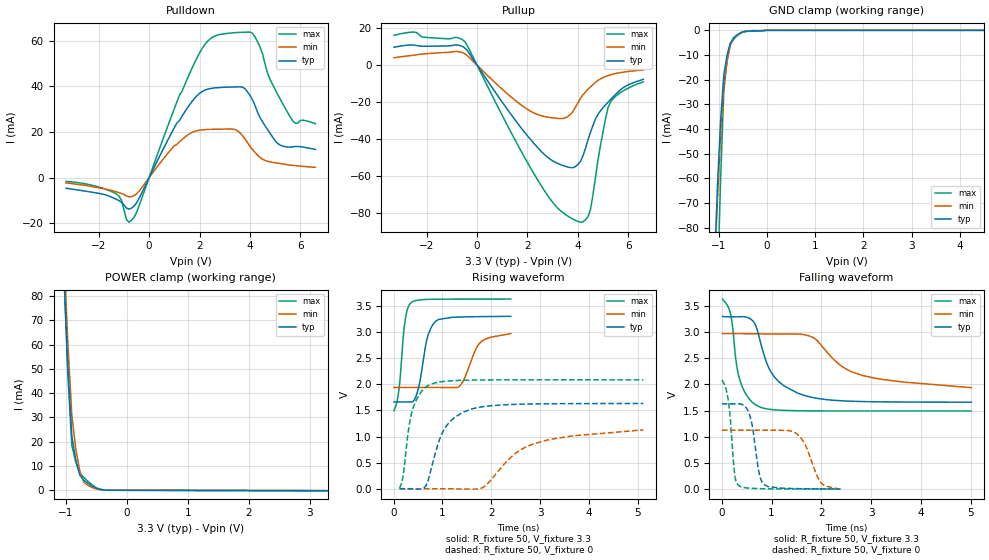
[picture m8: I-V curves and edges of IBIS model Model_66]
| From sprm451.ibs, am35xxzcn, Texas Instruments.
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| Model based on original model for BC1833DV50BTPBFHP18LL_7LM_X50
|   Sub model LL_7LM_X50_PU_ON_3P3
[model]   Model_66
|[Description]  3.3V-I/O-PU-X
|[Input Load]   PU
|[Output Drive]
|Voltage   3.3V
|Mode   I/O
Model_type   I/O
Polarity   Non-Inverting
Enable   Active-Low
Vinl =  0.8V
Vinh =  2V
Cref =  15pF
Rref =  100.0000M
Vref =  0V
Vmeas =  1.65
C_comp   1.683006p   1.492615p   1.787227p
[Model Spec]
Vinl   0.8V   0.8V   0.8V
Vinh   2V   2V   2V
[Temperature Range]   25   125   -40
[Voltage Range]   3.3   2.97   3.63
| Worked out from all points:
|   slope of the pulldown table from 0 to 0.495 V, typ, clamps not added: 44.5 ohm
|   slope of the pullup table from 0 to 0.495 V, typ, clamps not added: 49.1 ohm
|   GND clamp passes 1 mA (typ) near -0.54 V on its own axis
|   POWER clamp passes 1 mA (typ) near -0.51 V on its own axis
|   rising waveform, R_fixture 50, V_fixture 3.3: 20-80 % time 194ps typ, 279ps min, 122ps max; typ from 1.66 V to 3.3 V
|   rising waveform, R_fixture 50, V_fixture 0: 20-80 % time 424ps typ, 983ps min, 231ps max; typ from 0.004 V to 1.63 V
|   falling waveform, R_fixture 50, V_fixture 3.3: 20-80 % time 498ps typ, 965ps min, 226ps max; typ from 3.3 V to 1.66 V
|   falling waveform, R_fixture 50, V_fixture 0: 20-80 % time 155ps typ, 285ps min, 110ps max; typ from 1.63 V to 0.004 V
[POWER_clamp]
-3.3V     2.414A     2.856A     2.597A
-1.033V   91.31mA    100.7mA    91.95mA
-966.7mV  51.54mA    61.16mA    48.61mA
-900mV    22.22mA    30.81mA    18.41mA
-833.3mV  12.23mA    16.81mA    11.41mA
-766.7mV  6.164mA    7.579mA    7.005mA
-700mV    4.037mA    3.125mA    5.188mA
-566.7mV  1.798mA    1.149mA    2.234mA
-500mV    861.2uA    550uA      976.7uA
-433.3mV  389uA      264.1uA    415.9uA
-300mV    24.95uA    21.88uA    29.19uA
3.3V      -177.5uA   -135.7uA   -277.3uA
[Pulldown]
-3.3V     -4.669mA   -2.345mA   -1.683mA
-1.3V     -9.527mA   -6.237mA   -7.18mA
-900mV    -13.33mA   -8.044mA   -18.4mA
-700mV    -13.38mA   -8.364mA   -18.74mA
1.8V      34.72mA    20.23mA    50.28mA
2.3V      38.67mA    21.09mA    59.54mA
2.8V      39.47mA    21.22mA    62.74mA
3.5V      39.76mA    20.55mA    63.58mA
4.1V      34.11mA    12.32mA    63.3mA
5V        16.21mA    6.486mA    38.59mA
5.7V      13.47mA    5.354mA    24.85mA
6.6V      12.34mA    4.484mA    23.64mA
[Pullup]
-3.3V     9.738mA    4.045mA    16.21mA
-2.5V     10.91mA    5.432mA    17.94mA
-500mV    9.5mA      6.347mA    12.96mA
1.4V      -27.68mA   -17.82mA   -37.78mA
2.4V      -44.64mA   -26.76mA   -62.11mA
3.5V      -54.84mA   -28.6mA    -80.92mA
4.1V      -52.27mA   -18.13mA   -85.16mA
4.5V      -36.47mA   -11.82mA   -78.34mA
5V        -23.1mA    -6.724mA   -36.03mA
5.2V      -20.04mA   -5.652mA   -22.93mA
5.3V      -18.59mA   -5.203mA   -19.89mA
6.6V      -7.68mA    -2.683mA   -9.05mA
[GND_clamp]
-3.3V     -1.975A    -1.766A    -3.378A
-1.1V     -99.48mA   -100.9mA   -162.1mA
-1.033V   -63.84mA   -69.36mA   -106.2mA
-966.7mV  -36.69mA   -43.1mA    -60.36mA
-900mV    -18.03mA   -22.07mA   -24.57mA
-833.3mV  -10.17mA   -12.45mA   -12.64mA
-766.7mV  -5.227mA   -6.105mA   -5.683mA
-700mV    -3.195mA   -3.025mA   -3.716mA
-566.7mV  -1.239mA   -1.189mA   -1.328mA
-500mV    -580.8uA   -609.1uA   -631uA
-33.33mV  0A         0A         0A
6.6V      0A         0A         0A
[Ramp]
dV/dt_f 0.98252049/0.49548693n 0.61835083/0.96015548n  1.2814726/0.2246175n
dV/dt_r 0.98259665/0.42360656n 0.68007468/0.97384718n  1.2529846/0.23145552n
R_load = 50
[Rising Waveform]
R_fixture = 50
V_fixture = 3.3
V_fixture_min = 2.97
V_fixture_max = 3.63
4.168ps   1.662V     1.939V     1.494V
110.3ps   1.662V     1.939V     1.927V
233.1ps   1.662V     1.939V     3.214V
360.4ps   1.661V     1.939V     3.564V
500.2ps   1.902V     1.939V     3.61V
701.9ps   2.932V     1.939V     3.624V
872.4ps   3.214V     1.939V     3.627V
1.339ns   3.286V     1.955V     3.629V
1.773ns   3.294V     2.796V     3.63V
2.402ns   3.3V       2.97V      3.63V
[Rising Waveform]
R_fixture = 50
V_fixture = 0
V_fixture_min = 0
V_fixture_max = 0
118.8ps   4.128mV    2.524mV    5.94mV
189.8ps   4.131mV    2.524mV    231mV
373.5ps   1.933mV    2.524mV    1.472V
620.2ps   19.29mV    2.524mV    1.916V
735.5ps   263.4mV    2.524mV    1.99V
1.056ns   1.173V     2.538mV    2.059V
1.578ns   1.523V     -5.066mV   2.08V
1.857ns   1.576V     43.67mV    2.083V
2.836ns   1.624V     849.6mV    2.086V
5.119ns   1.634V     1.128V     2.086V
[Falling Waveform]
R_fixture = 50
V_fixture = 3.3
V_fixture_min = 2.97
V_fixture_max = 3.63
14.97ps   3.3V       2.97V      3.63V
177.6ps   3.292V     2.97V      3.335V
294.4ps   3.291V     2.97V      2.388V
370.9ps   3.293V     2.97V      2.058V
614.5ps   3.222V     2.969V     1.66V
733.1ps   2.967V     2.966V     1.583V
1.03ns    2.177V     2.964V     1.519V
1.611ns   1.806V     2.956V     1.498V
2.82ns    1.674V     2.175V     1.494V
5.015ns   1.662V     1.939V     1.494V
[Falling Waveform]
R_fixture = 50
V_fixture = 0
V_fixture_min = 0
V_fixture_max = 0
0s        1.634V     1.128V     2.086V
121.1ps   1.63V      1.128V     1.747V
259.8ps   1.63V      1.128V     275.4mV
347.3ps   1.63V      1.128V     67.2mV
564.9ps   1.398V     1.127V     20.71mV
749.5ps   312.3mV    1.126V     12.62mV
852.1ps   88.62mV    1.126V     9.874mV
1.492ns   13.75mV    1.07V      6.088mV
1.99ns    7.416mV    132.6mV    5.957mV
2.388ns   4.128mV    2.524mV    5.94mV
